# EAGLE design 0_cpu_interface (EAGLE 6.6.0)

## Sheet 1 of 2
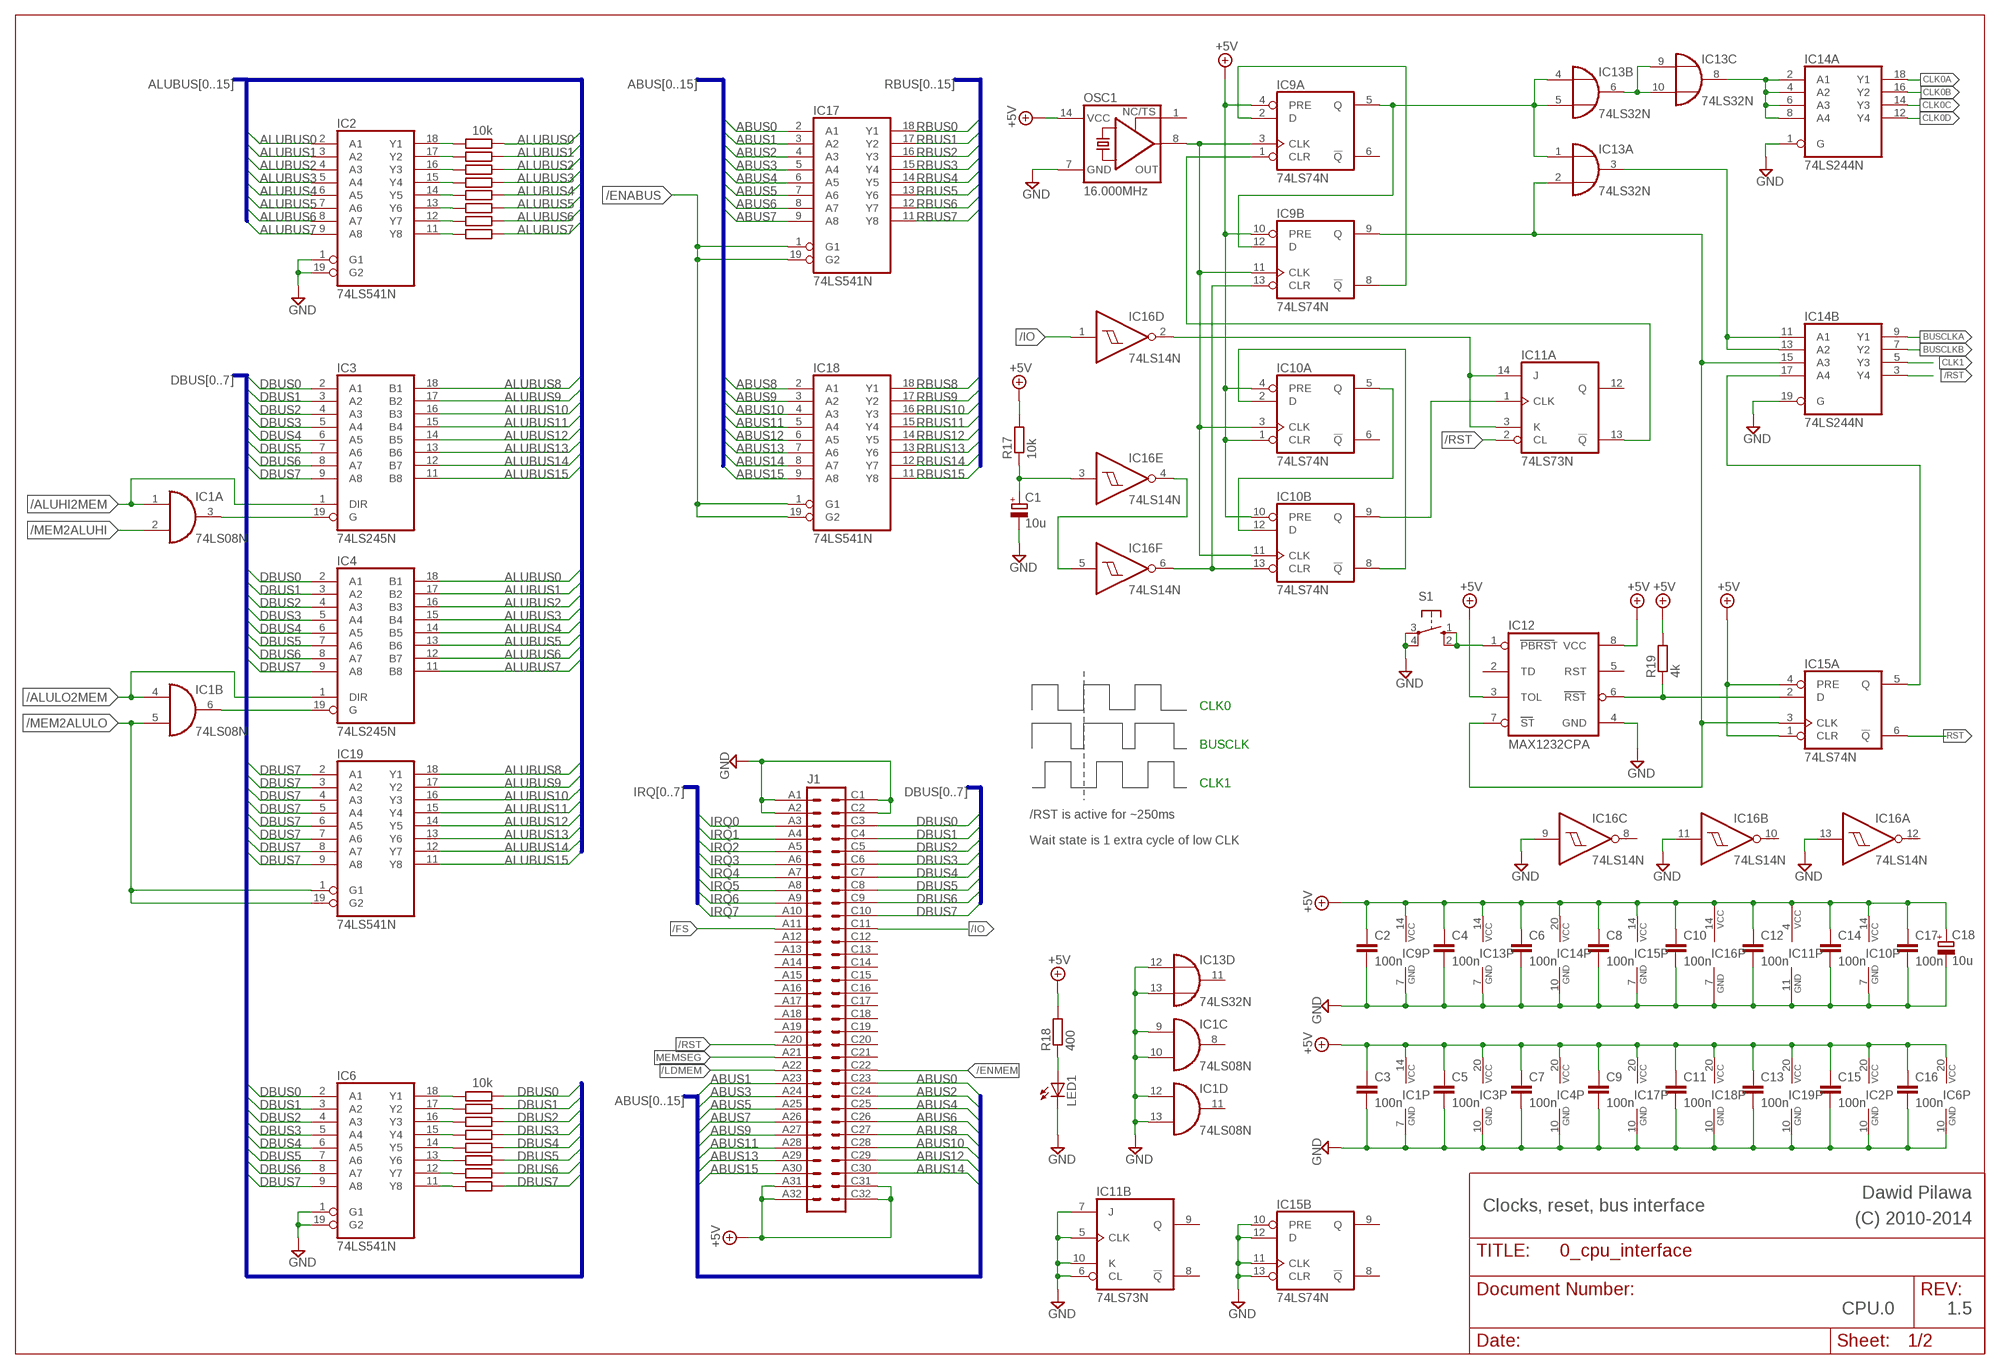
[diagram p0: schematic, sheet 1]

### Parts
C1  10u  CPOL-EUE2.5-5  [E2,5-5]
C2  100n  C-EU050-024X044  [C050-024X044]
C3  100n  C-EU050-024X044  [C050-024X044]
C4  100n  C-EU050-024X044  [C050-024X044]
C5  100n  C-EU050-024X044  [C050-024X044]
C6  100n  C-EU050-024X044  [C050-024X044]
C7  100n  C-EU050-024X044  [C050-024X044]
C8  100n  C-EU050-024X044  [C050-024X044]
C9  100n  C-EU050-024X044  [C050-024X044]
C10  100n  C-EU050-024X044  [C050-024X044]
C11  100n  C-EU050-024X044  [C050-024X044]
C12  100n  C-EU050-024X044  [C050-024X044]
C13  100n  C-EU050-024X044  [C050-024X044]
C14  100n  C-EU050-024X044  [C050-024X044]
C15  100n  C-EU050-024X044  [C050-024X044]
C16  100n  C-EU050-024X044  [C050-024X044]
C17  100n  C-EU050-024X044  [C050-024X044]
C18  10u  CPOL-EUE2.5-6  [E2,5-6]
IC1  74LS08N  [DIL14]
IC2  74LS541N  [DIL20]
IC3  74LS245N  [DIL20]
IC4  74LS245N  [DIL20]
IC6  74LS541N  [DIL20]
IC9  74LS74N  [DIL14]
IC10  74LS74N  [DIL14]
IC11  74LS73N  [DIL14]
IC12  MAX1232CPA  [DIL08]
IC13  74LS32N  [DIL14]
IC14  74LS244N  [DIL20]
IC15  74LS74N  [DIL14]
IC16  74LS14N  [DIL14]
IC17  74LS541N  [DIL20]
IC18  74LS541N  [DIL20]
IC19  74LS541N  [DIL20]
J1  VG64B  [VG64B]
LED1  LED5MM  [LED5MM]
OSC1  16.000MHz  XO-14  [DIL14S]
R1  10k  R-EU_0204/7  [0204/7]
R2  R-EU_0204/7  [0204/7]
R3  R-EU_0204/7  [0204/7]
R4  R-EU_0204/7  [0204/7]
R5  R-EU_0204/7  [0204/7]
R6  R-EU_0204/7  [0204/7]
R7  R-EU_0204/7  [0204/7]
R8  R-EU_0204/7  [0204/7]
R9  10k  R-EU_0204/7  [0204/7]
R10  R-EU_0204/7  [0204/7]
R11  R-EU_0204/7  [0204/7]
R12  R-EU_0204/7  [0204/7]
R13  R-EU_0204/7  [0204/7]
R14  R-EU_0204/7  [0204/7]
R15  R-EU_0204/7  [0204/7]
R16  R-EU_0204/7  [0204/7]
R17  10k  R-EU_0204/7  [0204/7]
R18  400  R-EU_0204/7  [0204/7]
R19  4k  R-EU_0204/7  [0204/7]
S1  10-XX  [B3F-10XX]

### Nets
+5V: C2.1 C3.1 C4.1 C5.1 C6.1 C7.1 C8.1 C9.1 C10.1 C11.1 C12.1 C13.1 C14.1 C15.1 C16.1 C17.1 C18.+ IC1.14(P:VCC) IC2.20(VCC) IC3.20(VCC) IC4.20(VCC) IC6.20(VCC) IC9.4(A:PRE) IC9.10(B:PRE) IC9.14(P:VCC) IC10.1(A:CLR) IC10.4(A:PRE) IC10.10(B:PRE) IC10.14(P:VCC) IC11.4(P:VCC) IC12.3(TOL) IC12.8(VCC) IC13.14(P:VCC) IC14.20(P:VCC) IC15.1(A:CLR) IC15.4(A:PRE) IC15.14(P:VCC) IC16.14(P:VCC) IC17.20(VCC) IC18.20(VCC) IC19.20(VCC) J1.A31 J1.A32 J1.C31 J1.C32 OSC1.14(VCC) R17.2 R18.2 R19.2 ; also sheet 2
/ALUHI2MEM: IC1.1(A:I0) IC3.1(DIR) ; also sheet 2
/ALULO2MEM: IC1.4(B:I0) IC4.1(DIR) ; also sheet 2
/ENABUS: IC17.1(G1) IC17.19(G2) IC18.1(G1) IC18.19(G2) ; also sheet 2
/ENMEM: J1.C22 ; also sheet 2
/FS: J1.A11 ; also sheet 2
/IO: IC16.1(D:I) J1.C11
/LDMEM: J1.A22 ; also sheet 2
/MEM2ALUHI: IC1.2(A:I1) ; also sheet 2
/MEM2ALULO: IC1.5(B:I1) IC19.1(G1) IC19.19(G2) ; also sheet 2
/RST: IC11.2(A:CL) IC14.3(B:Y4) J1.A20 ; also sheet 2
ABUS0: IC17.2(A1) J1.C23 ; also sheet 2
ABUS1: IC17.3(A2) J1.A23 ; also sheet 2
ABUS2: IC17.4(A3) J1.C24 ; also sheet 2
ABUS3: IC17.5(A4) J1.A24 ; also sheet 2
ABUS4: IC17.6(A5) J1.C25 ; also sheet 2
ABUS5: IC17.7(A6) J1.A25 ; also sheet 2
ABUS6: IC17.8(A7) J1.C26 ; also sheet 2
ABUS7: IC17.9(A8) J1.A26 ; also sheet 2
ABUS8: IC18.2(A1) J1.C27 ; also sheet 2
ABUS9: IC18.3(A2) J1.A27 ; also sheet 2
ABUS10: IC18.4(A3) J1.C28 ; also sheet 2
ABUS11: IC18.5(A4) J1.A28 ; also sheet 2
ABUS12: IC18.6(A5) J1.C29 ; also sheet 2
ABUS13: IC18.7(A6) J1.A29 ; also sheet 2
ABUS14: IC18.8(A7) J1.C30 ; also sheet 2
ABUS15: IC18.9(A8) J1.A30 ; also sheet 2
ALUBUS0: IC2.2(A1) IC4.18(B1) R1.2 ; also sheet 2
ALUBUS1: IC2.3(A2) IC4.17(B2) R2.2 ; also sheet 2
ALUBUS2: IC2.4(A3) IC4.16(B3) R3.2 ; also sheet 2
ALUBUS3: IC2.5(A4) IC4.15(B4) R4.2 ; also sheet 2
ALUBUS4: IC2.6(A5) IC4.14(B5) R5.2 ; also sheet 2
ALUBUS5: IC2.7(A6) IC4.13(B6) R6.2 ; also sheet 2
ALUBUS6: IC2.8(A7) IC4.12(B7) R7.2 ; also sheet 2
ALUBUS7: IC2.9(A8) IC4.11(B8) R8.2 ; also sheet 2
ALUBUS8: IC3.18(B1) IC19.18(Y1) ; also sheet 2
ALUBUS9: IC3.17(B2) IC19.17(Y2) ; also sheet 2
ALUBUS10: IC3.16(B3) IC19.16(Y3) ; also sheet 2
ALUBUS11: IC3.15(B4) IC19.15(Y4) ; also sheet 2
ALUBUS12: IC3.14(B5) IC19.14(Y5) ; also sheet 2
ALUBUS13: IC3.13(B6) IC19.13(Y6) ; also sheet 2
ALUBUS14: IC3.12(B7) IC19.12(Y7) ; also sheet 2
ALUBUS15: IC3.11(B8) IC19.11(Y8) ; also sheet 2
BUSCLK: IC13.3(A:O) IC14.11(B:A1) IC14.13(B:A2)
BUSCLKA: IC14.9(B:Y1) ; also sheet 2
BUSCLKB: IC14.7(B:Y2) ; also sheet 2
CLK0: IC9.5(A:Q) IC9.12(B:D) IC13.1(A:I0) IC13.4(B:I0) IC13.5(B:I1)
CLK0A: IC14.18(A:Y1) ; also sheet 2
CLK0B: IC14.16(A:Y2) ; also sheet 2
CLK0C: IC14.14(A:Y3) ; also sheet 2
CLK0D: IC14.12(A:Y4) ; also sheet 2
CLK1: IC14.5(B:Y3) ; also sheet 2
DBUS0: IC3.2(A1) IC4.2(A1) IC6.2(A1) J1.C3 R9.2 ; also sheet 2
DBUS1: IC3.3(A2) IC4.3(A2) IC6.3(A2) J1.C4 R10.2 ; also sheet 2
DBUS2: IC3.4(A3) IC4.4(A3) IC6.4(A3) J1.C5 R11.2 ; also sheet 2
DBUS3: IC3.5(A4) IC4.5(A4) IC6.5(A4) J1.C6 R12.2 ; also sheet 2
DBUS4: IC3.6(A5) IC4.6(A5) IC6.6(A5) J1.C7 R13.2 ; also sheet 2
DBUS5: IC3.7(A6) IC4.7(A6) IC6.7(A6) J1.C8 R14.2 ; also sheet 2
DBUS6: IC3.8(A7) IC4.8(A7) IC6.8(A7) J1.C9 R15.2 ; also sheet 2
DBUS7: IC3.9(A8) IC4.9(A8) IC6.9(A8) IC19.2(A1) IC19.3(A2) IC19.4(A3) IC19.5(A4) IC19.6(A5) IC19.7(A6) IC19.8(A7) IC19.9(A8) J1.C10 R16.2 ; also sheet 2
GND: C1.- C2.2 C3.2 C4.2 C5.2 C6.2 C7.2 C8.2 C9.2 C10.2 C11.2 C12.2 C13.2 C14.2 C15.2 C16.2 C17.2 C18.- IC1.7(P:GND) IC1.9(C:I0) IC1.10(C:I1) IC1.12(D:I0) IC1.13(D:I1) IC2.1(G1) IC2.10(GND) IC2.19(G2) IC3.10(GND) IC4.10(GND) IC6.1(G1) IC6.10(GND) IC6.19(G2) IC9.7(P:GND) IC10.7(P:GND) IC11.5(B:CLK) IC11.6(B:CL) IC11.7(B:J) IC11.10(B:K) IC11.11(P:GND) IC12.4(GND) IC13.7(P:GND) IC13.12(D:I0) IC13.13(D:I1) IC14.1(A:G) IC14.10(P:GND) IC14.19(B:G) IC15.7(P:GND) IC15.10(B:PRE) IC15.11(B:CLK) IC15.12(B:D) IC15.13(B:CLR) IC16.7(P:GND) IC16.9(C:I) IC16.11(B:I) IC16.13(A:I) IC17.10(GND) IC18.10(GND) IC19.10(GND) J1.A1 J1.A2 J1.C1 J1.C2 LED1.K(C) OSC1.7(GND) S1.3(P) S1.4(P1) ; also sheet 2
IRQ0: J1.A3 ; also sheet 2
IRQ1: J1.A4 ; also sheet 2
IRQ2: J1.A5 ; also sheet 2
IRQ3: J1.A6 ; also sheet 2
IRQ4: J1.A7 ; also sheet 2
IRQ5: J1.A8 ; also sheet 2
IRQ6: J1.A9 ; also sheet 2
IRQ7: J1.A10 ; also sheet 2
MEMSEG: J1.A21 ; also sheet 2
N$1: IC1.3(A:O) IC3.19(G)
N$2: IC1.6(B:O) IC4.19(G)
N$3: IC2.18(Y1) R1.1
N$4: IC2.17(Y2) R2.1
N$5: IC2.16(Y3) R3.1
N$6: IC2.15(Y4) R4.1
N$7: IC2.14(Y5) R5.1
N$8: IC2.13(Y6) R6.1
N$9: IC2.12(Y7) R7.1
N$10: IC2.11(Y8) R8.1
N$11: IC6.18(Y1) R9.1
N$12: IC6.17(Y2) R10.1
N$13: IC6.16(Y3) R11.1
N$14: IC6.15(Y4) R12.1
N$15: IC6.14(Y5) R13.1
N$16: IC6.12(Y7) R15.1
N$17: IC6.11(Y8) R16.1
N$18: IC6.13(Y6) R14.1
N$19: IC12.1(PBRST) S1.1(S) S1.2(S1)
N$20: IC9.3(A:CLK) IC9.11(B:CLK) IC10.3(A:CLK) IC10.11(B:CLK) OSC1.8(OUT)
N$21: LED1.A R18.1
N$22: IC9.2(A:D) IC9.8(B:!Q)
N$23: IC14.17(B:A4) IC15.5(A:Q)
N$24: IC12.6(RST) IC15.2(A:D) R19.1
N$25: IC10.2(A:D) IC10.8(B:!Q)
N$26: IC13.8(C:O) IC14.2(A:A1) IC14.4(A:A2) IC14.6(A:A3) IC14.8(A:A4)
N$27: IC9.1(A:CLR) IC11.13(A:!Q)
N$28: C1.+ IC16.3(E:I) R17.1
N$29: IC13.6(B:O) IC13.9(C:I0) IC13.10(C:I1)
N$30: IC9.9(B:Q) IC12.7(ST) IC13.2(A:I1) IC14.15(B:A3) IC15.3(A:CLK)
N$31: IC10.5(A:Q) IC10.12(B:D)
N$32: IC10.9(B:Q) IC11.1(A:CLK)
N$33: IC11.3(A:K) IC11.14(A:J) IC16.2(D:O)
N$34: IC16.4(E:O) IC16.5(F:I)
N$35: IC9.13(B:CLR) IC10.13(B:CLR) IC16.6(F:O)
RBUS0: IC17.18(Y1) ; also sheet 2
RBUS1: IC17.17(Y2) ; also sheet 2
RBUS2: IC17.16(Y3) ; also sheet 2
RBUS3: IC17.15(Y4) ; also sheet 2
RBUS4: IC17.14(Y5) ; also sheet 2
RBUS5: IC17.13(Y6) ; also sheet 2
RBUS6: IC17.12(Y7) ; also sheet 2
RBUS7: IC17.11(Y8) ; also sheet 2
RBUS8: IC18.18(Y1) ; also sheet 2
RBUS9: IC18.17(Y2) ; also sheet 2
RBUS10: IC18.16(Y3) ; also sheet 2
RBUS11: IC18.15(Y4) ; also sheet 2
RBUS12: IC18.14(Y5) ; also sheet 2
RBUS13: IC18.13(Y6) ; also sheet 2
RBUS14: IC18.12(Y7) ; also sheet 2
RBUS15: IC18.11(Y8) ; also sheet 2
RST: IC15.6(A:!Q) ; also sheet 2
Unconnected: IC1.8(C:O) IC1.11(D:O) IC9.6(A:!Q) IC10.6(A:!Q) IC11.8(B:!Q) IC11.9(B:Q) IC11.12(A:Q) IC12.2(TD) IC12.5(RST) IC13.11(D:O) IC15.8(B:!Q) IC15.9(B:Q) IC16.8(C:O) IC16.10(B:O) IC16.12(A:O) J1.A12 J1.A13 J1.A14 J1.A15 J1.A16 J1.A17 J1.A18 J1.A19 J1.C12 J1.C13 J1.C14 J1.C15 J1.C16 J1.C17 J1.C18 J1.C19 J1.C20 J1.C21 OSC1.1(TS)

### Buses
DBUS[0..7]
ALUBUS[0..15]
RBUS[0..15]
IRQ[0..7]
ABUS[0..15]

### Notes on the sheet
- CLK0
- BUSCLK
- CLK1
- /RST is active for ~250ms
- Wait state is 1 extra cycle of low CLK
- Dawid Pilawa
- Clocks, reset, bus interface | (C) 2010-2014
- CPU.0 | 1.5

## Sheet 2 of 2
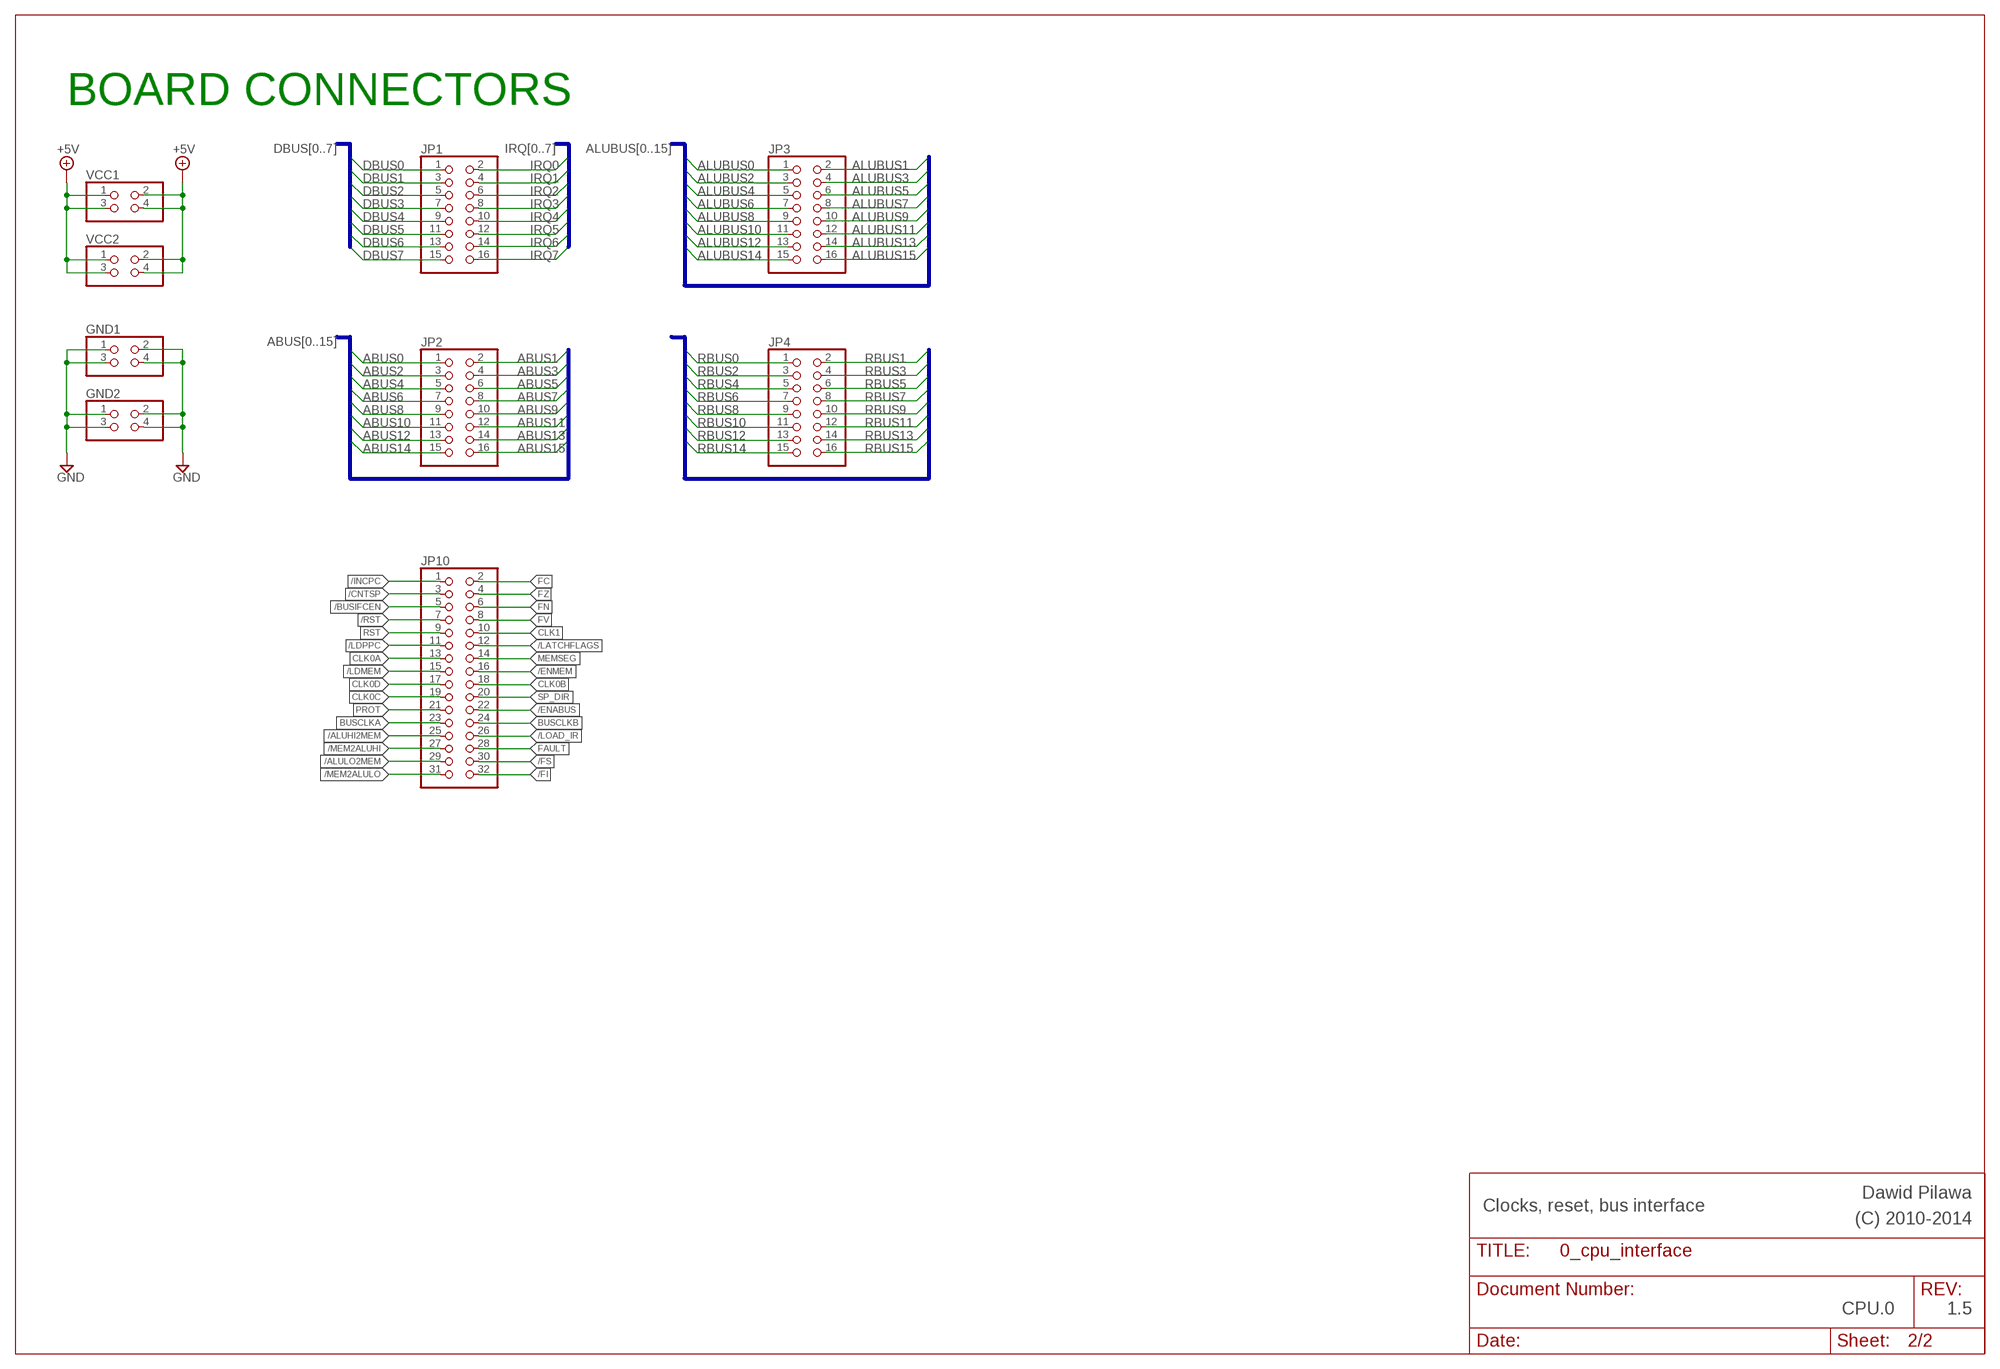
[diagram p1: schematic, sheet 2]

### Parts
GND1  PINHD-2X2  [2X02]
GND2  PINHD-2X2  [2X02]
JP1  PINHD-2X8  [2X08]
JP2  PINHD-2X8  [2X08]
JP3  PINHD-2X8  [2X08]
JP4  PINHD-2X8  [2X08]
JP10  PINHD-2X16  [2X16]
VCC1  PINHD-2X2  [2X02]
VCC2  PINHD-2X2  [2X02]

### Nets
+5V: VCC1.1 VCC1.2 VCC1.3 VCC1.4 VCC2.1 VCC2.2 VCC2.3 VCC2.4 ; also sheet 1
/ALUHI2MEM: JP10.25 ; also sheet 1
/ALULO2MEM: JP10.29 ; also sheet 1
/BUSIFCEN: JP10.5
/CNTSP: JP10.3
/ENABUS: JP10.22 ; also sheet 1
/ENMEM: JP10.16 ; also sheet 1
/FI: JP10.32
/FS: JP10.30 ; also sheet 1
/INCPC: JP10.1
/LATCHFLAGS: JP10.12
/LDMEM: JP10.15 ; also sheet 1
/LDPPC: JP10.11
/LOAD_IR: JP10.26
/MEM2ALUHI: JP10.27 ; also sheet 1
/MEM2ALULO: JP10.31 ; also sheet 1
/RST: JP10.7 ; also sheet 1
ABUS0: JP2.1 ; also sheet 1
ABUS1: JP2.2 ; also sheet 1
ABUS2: JP2.3 ; also sheet 1
ABUS3: JP2.4 ; also sheet 1
ABUS4: JP2.5 ; also sheet 1
ABUS5: JP2.6 ; also sheet 1
ABUS6: JP2.7 ; also sheet 1
ABUS7: JP2.8 ; also sheet 1
ABUS8: JP2.9 ; also sheet 1
ABUS9: JP2.10 ; also sheet 1
ABUS10: JP2.11 ; also sheet 1
ABUS11: JP2.12 ; also sheet 1
ABUS12: JP2.13 ; also sheet 1
ABUS13: JP2.14 ; also sheet 1
ABUS14: JP2.15 ; also sheet 1
ABUS15: JP2.16 ; also sheet 1
ALUBUS0: JP3.1 ; also sheet 1
ALUBUS1: JP3.2 ; also sheet 1
ALUBUS2: JP3.3 ; also sheet 1
ALUBUS3: JP3.4 ; also sheet 1
ALUBUS4: JP3.5 ; also sheet 1
ALUBUS5: JP3.6 ; also sheet 1
ALUBUS6: JP3.7 ; also sheet 1
ALUBUS7: JP3.8 ; also sheet 1
ALUBUS8: JP3.9 ; also sheet 1
ALUBUS9: JP3.10 ; also sheet 1
ALUBUS10: JP3.11 ; also sheet 1
ALUBUS11: JP3.12 ; also sheet 1
ALUBUS12: JP3.13 ; also sheet 1
ALUBUS13: JP3.14 ; also sheet 1
ALUBUS14: JP3.15 ; also sheet 1
ALUBUS15: JP3.16 ; also sheet 1
BUSCLKA: JP10.23 ; also sheet 1
BUSCLKB: JP10.24 ; also sheet 1
CLK0A: JP10.13 ; also sheet 1
CLK0B: JP10.18 ; also sheet 1
CLK0C: JP10.19 ; also sheet 1
CLK0D: JP10.17 ; also sheet 1
CLK1: JP10.10 ; also sheet 1
DBUS0: JP1.1 ; also sheet 1
DBUS1: JP1.3 ; also sheet 1
DBUS2: JP1.5 ; also sheet 1
DBUS3: JP1.7 ; also sheet 1
DBUS4: JP1.9 ; also sheet 1
DBUS5: JP1.11 ; also sheet 1
DBUS6: JP1.13 ; also sheet 1
DBUS7: JP1.15 ; also sheet 1
FAULT: JP10.28
FC: JP10.2
FN: JP10.6
FV: JP10.8
FZ: JP10.4
GND: GND1.1 GND1.2 GND1.3 GND1.4 GND2.1 GND2.2 GND2.3 GND2.4 ; also sheet 1
IRQ0: JP1.2 ; also sheet 1
IRQ1: JP1.4 ; also sheet 1
IRQ2: JP1.6 ; also sheet 1
IRQ3: JP1.8 ; also sheet 1
IRQ4: JP1.10 ; also sheet 1
IRQ5: JP1.12 ; also sheet 1
IRQ6: JP1.14 ; also sheet 1
IRQ7: JP1.16 ; also sheet 1
MEMSEG: JP10.14 ; also sheet 1
PROT: JP10.21
RBUS0: JP4.1 ; also sheet 1
RBUS1: JP4.2 ; also sheet 1
RBUS2: JP4.3 ; also sheet 1
RBUS3: JP4.4 ; also sheet 1
RBUS4: JP4.5 ; also sheet 1
RBUS5: JP4.6 ; also sheet 1
RBUS6: JP4.7 ; also sheet 1
RBUS7: JP4.8 ; also sheet 1
RBUS8: JP4.9 ; also sheet 1
RBUS9: JP4.10 ; also sheet 1
RBUS10: JP4.11 ; also sheet 1
RBUS11: JP4.12 ; also sheet 1
RBUS12: JP4.13 ; also sheet 1
RBUS13: JP4.14 ; also sheet 1
RBUS14: JP4.15 ; also sheet 1
RBUS15: JP4.16 ; also sheet 1
RST: JP10.9 ; also sheet 1
SP_DIR: JP10.20

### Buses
DBUS[0..7]
ALUBUS[0..15]
RBUS[0..15]
IRQ[0..7]
ABUS[0..15]

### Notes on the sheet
- BOARD CONNECTORS
- Dawid Pilawa
- Clocks, reset, bus interface | (C) 2010-2014
- CPU.0 | 1.5

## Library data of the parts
C1 C18 = rcl:CPOL-EU: POLARIZED CAPACITOR, European symbol
C2-C17 = rcl:C-EU: CAPACITOR, European symbol
GND1 GND2 VCC1 VCC2 = pinhead:PINHD-2X2: PIN HEADER
IC1 = 74xx-eu:74*08: Quad 2-input AND gate
IC2 IC6 IC17-IC19 = 74xx-eu:74*541: Octal BUFFER and LINE DRIVER, 3-state
IC3 IC4 = 74xx-eu:74*245: Octal BUS TRANSCEIVER, 3-state
IC9 IC10 IC15 = 74xx-eu:74*74: Dual D type positive edge triggered FLIP FLOP, preset and clear
IC11 = 74xx-us:74*73: Dual J-K FLIP FLOP, clear
IC12 = maxim:MAX1232CPA: MONITOR DEVICE
IC13 = 74xx-eu:74*32: Quad 2-input OR gate
IC14 = 74xx-eu:74*244: Octal BUFFER and LINE DRIVER, 3-state
IC16 = 74xx-us:74*14: Hex schmitt trigger INVERTER
J1 = 19inch:VG64: PCB EUROCARD, 64-pin type C/AC, 2.54 mm
JP1-JP4 = pinhead:PINHD-2X8: PIN HEADER
JP10 = pinhead:PINHD-2X16: PIN HEADER
LED1 = led:LED: LED
OSC1 = crystal:XO-: CRYSTAL
R1-R19 = rcl:R-EU_: RESISTOR, European symbol
S1 = switch-omron:10-XX: OMRON SWITCH

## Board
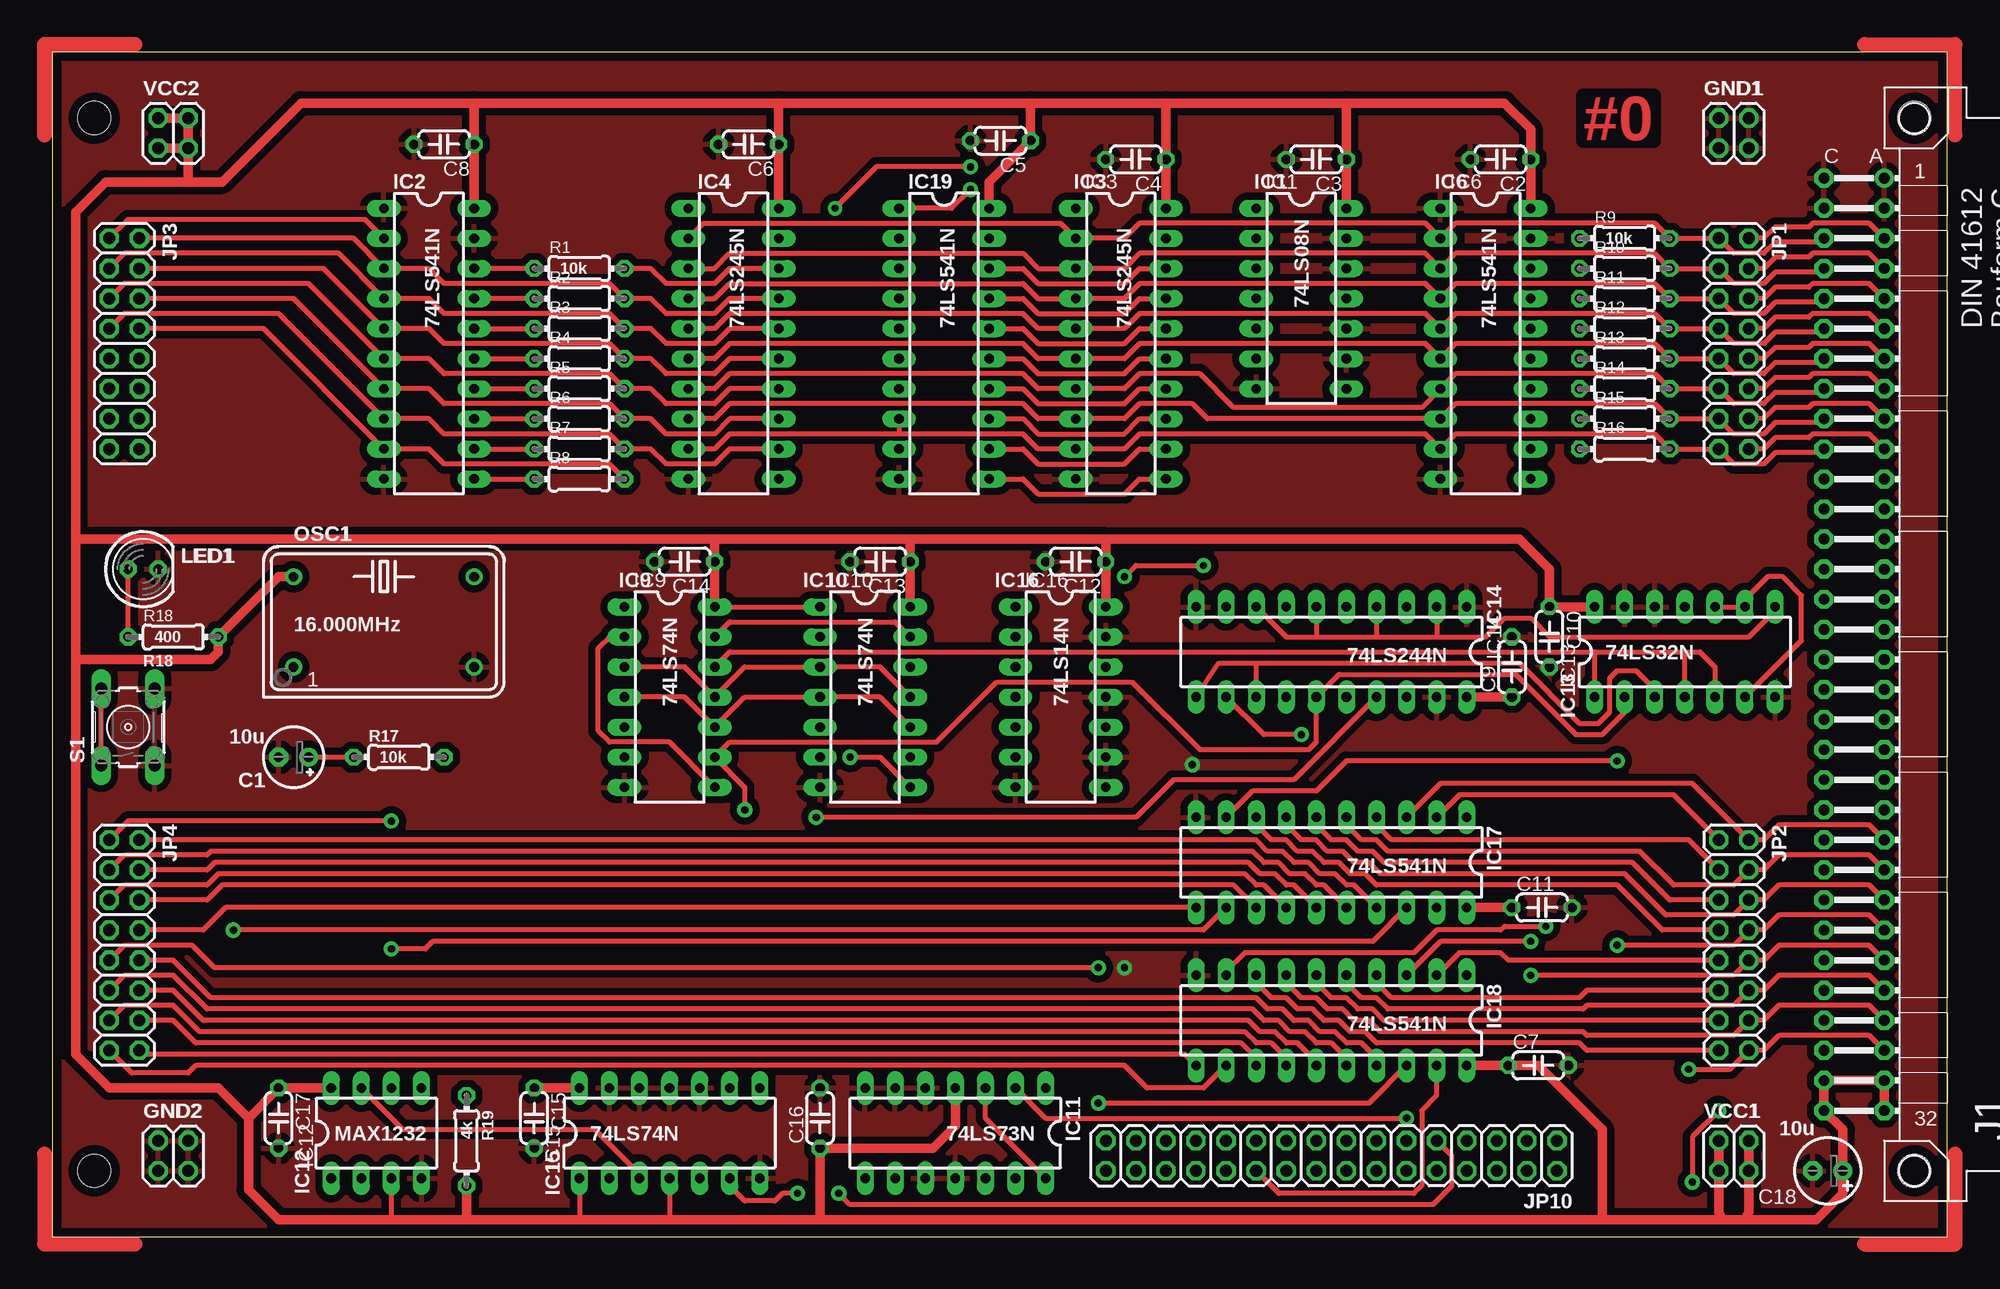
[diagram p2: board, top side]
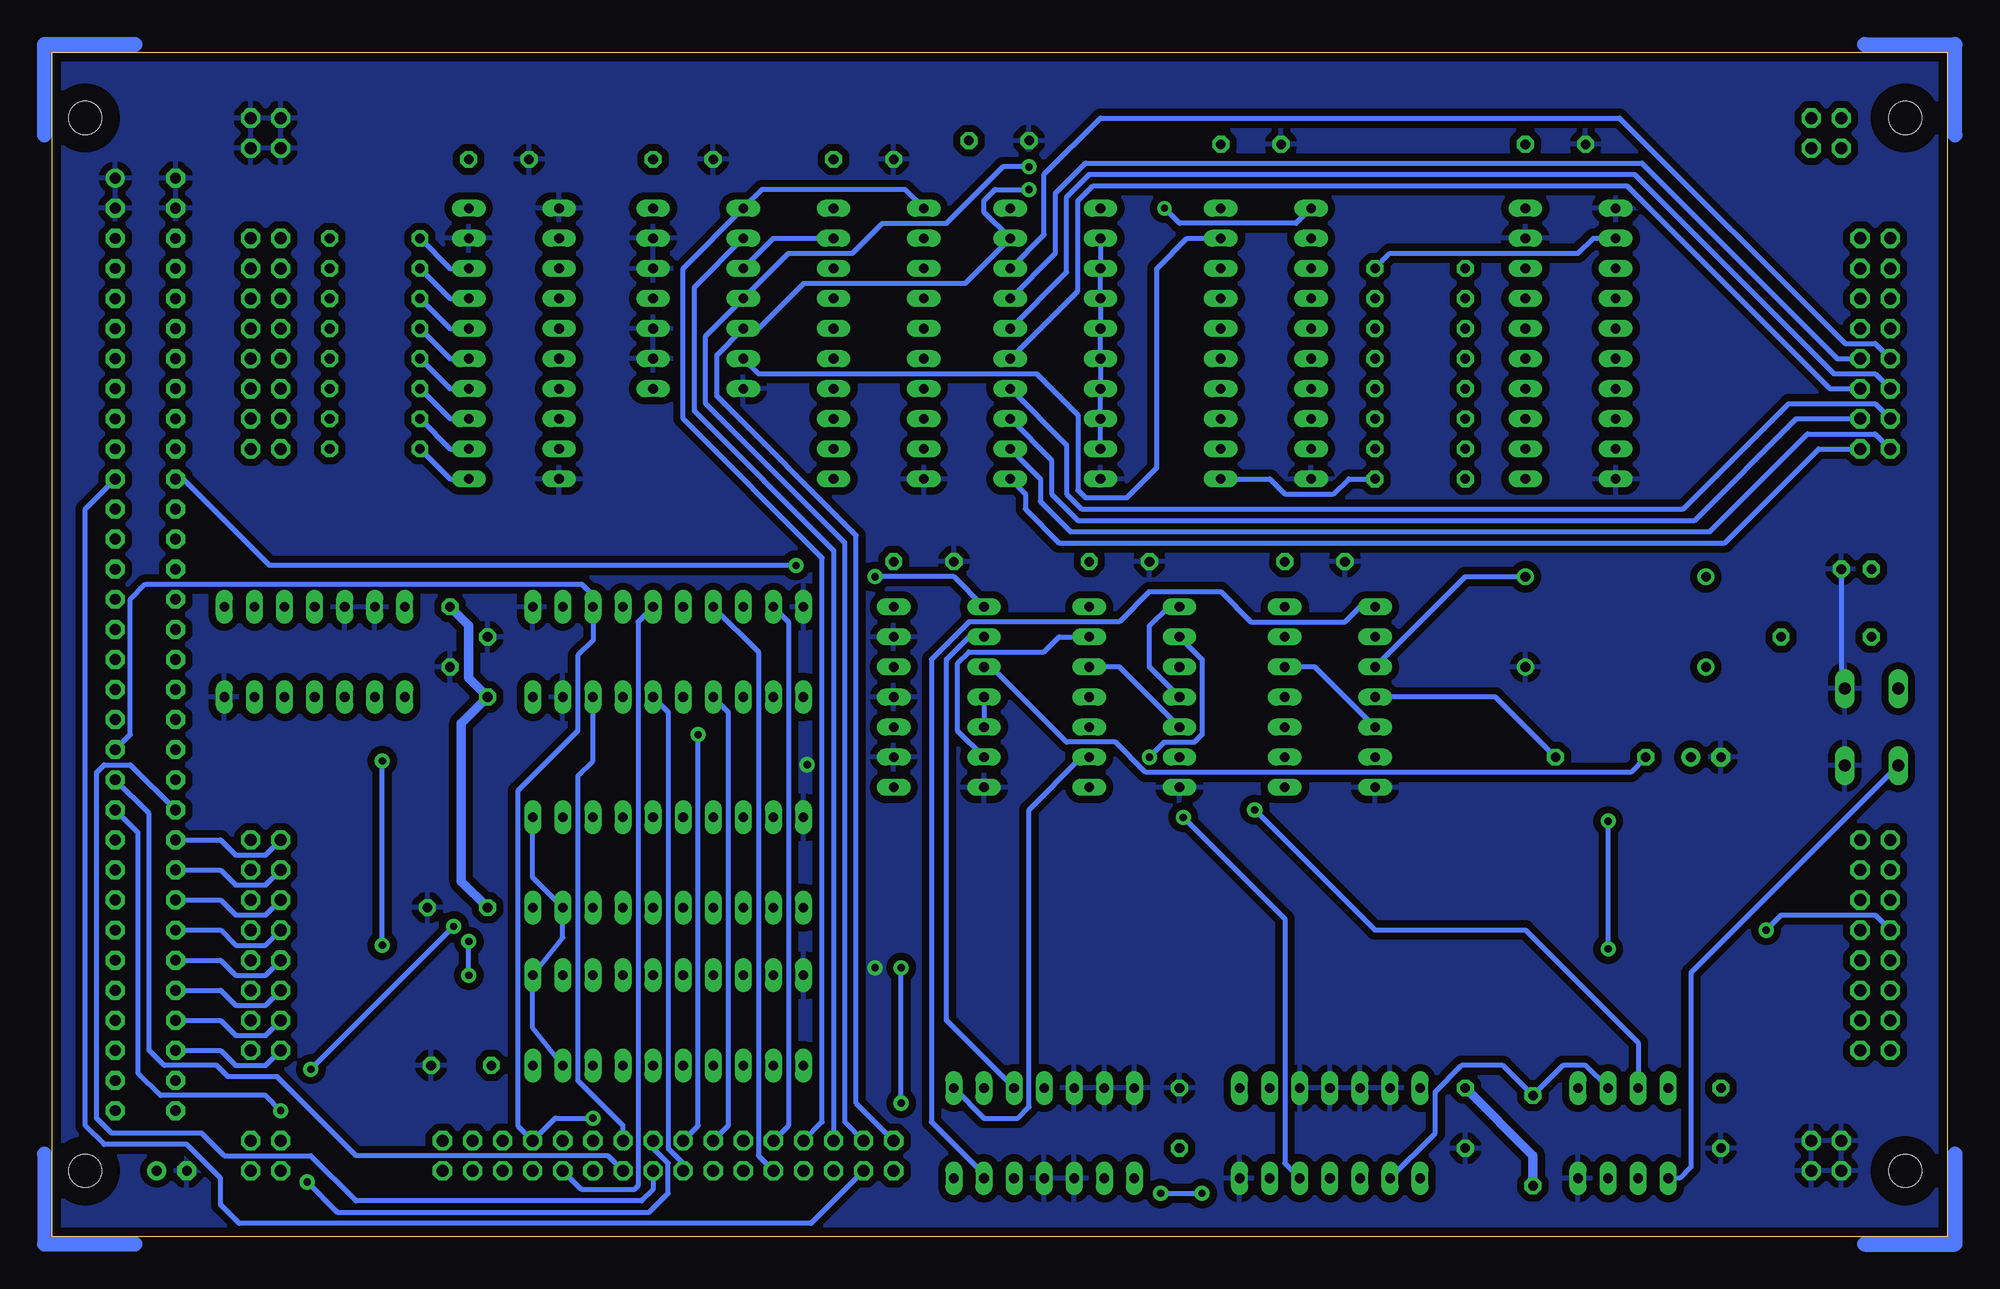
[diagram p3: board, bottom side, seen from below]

Size 160.02 x 100.03 mm. Coordinates in mm from the lower left corner, seen from the top.
Copper layers (1*16): Top 0.035mm / dielectric 1.5mm / Bottom 0.035mm
Design rules "homebrew_pcb": minimum track width 16mil, minimum drill 24mil, track to track 16mil, track to pad 10mil, pad to pad 10mil, via to via 10mil, smd to smd 8mil, copper to edge 30mil, drill to drill 10mil, minimum pad ring 12mil, minimum via ring 12mil, stop-mask expansion 4mil, vias tented up to drill 0mil, thermal gap 24mil

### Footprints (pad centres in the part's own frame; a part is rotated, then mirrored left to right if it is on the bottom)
E2,5-5 = drill 0.813 pad 1.6: + -1.27,0 | drill 0.813 pad 1.6 octagon: - 1.27,0
C050-024X044 = drill 0.813 octagon: 1 -2.54,0; 2 2.54,0
E2,5-6 = drill 0.813 pad 1.6: + -1.27,0 | drill 0.813 pad 1.6 octagon: - 1.27,0
2X02 = drill 1.016 octagon: 1 -1.27,-1.27; 2 -1.27,1.27; 3 1.27,-1.27; 4 1.27,1.27
DIL14 = drill 0.813 long: 1 -7.62,-3.81; 2 -5.08,-3.81; 3 -2.54,-3.81; 4 0,-3.81; 5 2.54,-3.81; 6 5.08,-3.81; 7 7.62,-3.81; 8 7.62,3.81; 9 5.08,3.81; 10 2.54,3.81; 11 0,3.81; 12 -2.54,3.81; 13 -5.08,3.81; 14 -7.62,3.81
DIL20 = drill 0.813 long: 1 -11.43,-3.81; 2 -8.89,-3.81; 3 -6.35,-3.81; 4 -3.81,-3.81; 5 -1.27,-3.81; 6 1.27,-3.81; 7 3.81,-3.81; 8 6.35,-3.81; 9 8.89,-3.81; 10 11.43,-3.81; 11 11.43,3.81; 12 8.89,3.81; 13 6.35,3.81; 14 3.81,3.81; 15 1.27,3.81; 16 -1.27,3.81; 17 -3.81,3.81; 18 -6.35,3.81; 19 -8.89,3.81; 20 -11.43,3.81
DIL08 = drill 0.813 long: 1 -3.81,-3.81; 2 -1.27,-3.81; 3 1.27,-3.81; 4 3.81,-3.81; 5 3.81,3.81; 6 1.27,3.81; 7 -1.27,3.81; 8 -3.81,3.81
VG64B = drill 0.914 pad 1.6: A1 154.94,39.37 | drill 0.914 pad 1.6 octagon: A2 154.94,36.83; A3 154.94,34.29; A4 154.94,31.75; A5 154.94,29.21; A6 154.94,26.67; A7 154.94,24.13; A8 154.94,21.59; A9 154.94,19.05; A10 154.94,16.51; A11 154.94,13.97; A12 154.94,11.43; A13 154.94,8.89; A14 154.94,6.35; A15 154.94,3.81; A16 154.94,1.27; A17 154.94,-1.27; A18 154.94,-3.81; A19 154.94,-6.35; A20 154.94,-8.89; A21 154.94,-11.43; A22 154.94,-13.97; A23 154.94,-16.51; A24 154.94,-19.05; A25 154.94,-21.59; A26 154.94,-24.13; A27 154.94,-26.67; A28 154.94,-29.21; A29 154.94,-31.75; A30 154.94,-34.29; A31 154.94,-36.83; A32 154.94,-39.37; C1 149.86,39.37; C2 149.86,36.83; C3 149.86,34.29; C4 149.86,31.75; C5 149.86,29.21; C6 149.86,26.67; C7 149.86,24.13; C8 149.86,21.59; C9 149.86,19.05; C10 149.86,16.51; C11 149.86,13.97; C12 149.86,11.43; C13 149.86,8.89; C14 149.86,6.35; C15 149.86,3.81; C16 149.86,1.27; C17 149.86,-1.27; C18 149.86,-3.81; C19 149.86,-6.35; C20 149.86,-8.89; C21 149.86,-11.43; C22 149.86,-13.97; C23 149.86,-16.51; C24 149.86,-19.05; C25 149.86,-21.59; C26 149.86,-24.13; C27 149.86,-26.67; C28 149.86,-29.21; C29 149.86,-31.75; C30 149.86,-34.29; C31 149.86,-36.83; C32 149.86,-39.37 | hole 2.794: 157.48,44.45; 157.48,-44.45; 3.81,-44.45; 3.81,44.45
2X08 = drill 1.016 octagon: 1 -8.89,-1.27; 2 -8.89,1.27; 3 -6.35,-1.27; 4 -6.35,1.27; 5 -3.81,-1.27; 6 -3.81,1.27; 7 -1.27,-1.27; 8 -1.27,1.27; 9 1.27,-1.27; 10 1.27,1.27; 11 3.81,-1.27; 12 3.81,1.27; 13 6.35,-1.27; 14 6.35,1.27; 15 8.89,-1.27; 16 8.89,1.27
2X16 = drill 1.016 octagon: 1 -19.05,-1.27; 2 -19.05,1.27; 3 -16.51,-1.27; 4 -16.51,1.27; 5 -13.97,-1.27; 6 -13.97,1.27; 7 -11.43,-1.27; 8 -11.43,1.27; 9 -8.89,-1.27; 10 -8.89,1.27; 11 -6.35,-1.27; 12 -6.35,1.27; 13 -3.81,-1.27; 14 -3.81,1.27; 15 -1.27,-1.27; 16 -1.27,1.27; 17 1.27,-1.27; 18 1.27,1.27; 19 3.81,-1.27; 20 3.81,1.27; 21 6.35,-1.27; 22 6.35,1.27; 23 8.89,-1.27; 24 8.89,1.27; 25 11.43,-1.27; 26 11.43,1.27; 27 13.97,-1.27; 28 13.97,1.27; 29 16.51,-1.27; 30 16.51,1.27; 31 19.05,-1.27; 32 19.05,1.27
LED5MM = drill 0.813 octagon: A -1.27,0; K 1.27,0
DIL14S = drill 0.813: 1 -7.62,-3.81; 7 7.62,-3.81; 8 7.62,3.81; 14 -7.62,3.81
0204/7 = drill 0.813 octagon: 1 -3.81,0; 2 3.81,0
B3F-10XX = drill 1.016 long: 1 -3.251,2.261; 2 3.251,2.261; 3 -3.251,-2.261; 4 3.251,-2.261

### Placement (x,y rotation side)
C1  20.38,40.49 180 top
C2  122.3,90.97 180 top
C3  106.74,90.97 180 top
C4  91.5,90.97 180 top
C5  80.07,92.56 180 top
C6  58.8,92.24 180 top
C7  125.48,14.45 0 top
C8  33.08,92.24 180 top
C9  123.25,48.11 90 top
C10  126.43,50.65 270 top
C11  125.79,27.79 0 top
C12  86.42,57 180 top
C13  69.91,57 180 top
C14  53.4,57 180 top
C15  40.7,10.01 270 top
C16  64.83,10.01 90 top
C17  19.11,10.01 270 top
C18  149.92,5.56 180 top
GND1  141.99,93.19 0 top
GND2  10.22,6.83 0 top
IC1  105.47,79.22 270 top
IC2  31.81,75.41 270 top
IC3  90.23,75.41 270 top
IC4  57.53,75.41 270 top
IC6  121.03,75.41 270 top
IC9  52.13,45.57 270 top
IC10  68.64,45.57 270 top
IC11  76.26,8.74 180 top
IC12  27.37,8.74 0 top
IC13  137.86,49.38 0 top
IC14  108.01,49.38 180 top
IC15  52.13,8.74 0 top
IC16  85.15,45.57 270 top
IC17  108.01,31.6 180 top
IC18  108.01,18.26 180 top
IC19  75.31,75.41 270 top
J1  -0.25,50.01 0 top
JP1  141.99,75.41 270 top
JP2  141.99,24.61 270 top
JP3  6.1,75.41 270 top
JP4  6.1,24.61 270 top
JP10  108.01,6.83 180 top
LED1  7.68,56.36 0 top
OSC1  28,51.92 0 top
R1  44.51,81.76 0 top
R2  44.51,79.22 0 top
R3  44.51,76.68 0 top
R4  44.51,74.14 0 top
R5  44.51,71.6 0 top
R6  44.51,69.06 0 top
R7  44.51,66.52 0 top
R8  44.51,63.98 0 top
R9  132.78,84.3 0 top
R10  132.78,81.76 0 top
R11  132.78,79.22 0 top
R12  132.78,76.68 0 top
R13  132.78,74.14 0 top
R14  132.78,71.6 0 top
R15  132.78,69.06 0 top
R16  132.78,66.52 0 top
R17  29.27,40.49 0 top
R18  10.22,50.65 0 top
R19  34.99,8.1 270 top
S1  6.41,43.03 90 top
VCC1  141.99,6.83 0 top
VCC2  10.22,93.19 0 top

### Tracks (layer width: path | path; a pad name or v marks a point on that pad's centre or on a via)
+5V
  Top 0.406: IC12.3 28.64,1.43 | IC15.1 44.51,1.43 | IC15.4 52.13,1.43 | IC10.10 69.91,45.57 IC10.4 58.48,45.57 IC9.10 53.4,45.57 IC9.4 | IC9.14 IC10.1
  Top 0.813: 130.87,1.43 64.83,1.43 | 64.83,1.43 52.13,1.43 44.51,1.43 34.99,1.43 | 34.99,1.43 28.64,1.43 19.11,1.43 16.57,3.98 16.57,10.01 | 1.97,48.74 1.97,58.9 | 1.97,58.9 1.97,86.52 4.51,89.07 11.49,89.07 | 35.62,95.73 21.02,95.73 14.35,89.07 11.49,89.07 | 35.62,95.73 61.34,95.73 | 61.34,95.73 82.61,95.73 | 82.61,95.73 94.04,95.73 | 94.04,95.73 109.28,95.73 | 109.28,95.73 122.62,95.73 124.84,93.51 C2.1 IC6.20 | 109.28,95.73 C3.1 IC1.14 | 94.04,95.73 C4.1 IC3.20 | 88.96,58.9 72.45,58.9 | 72.45,58.9 55.94,58.9 | 55.94,58.9 1.97,58.9 | 88.96,58.9 C12.1 IC16.14 | 72.45,58.9 C13.1 IC10.14 | 55.94,58.9 C14.1 IC9.14 | OSC1.14 19.11,55.73 R18.2 14.03,49.38 13.4,48.74 1.97,48.74 | IC15.14 C15.1 | IC12.8 C17.1 16.57,10.01 | 64.83,1.43 C16.1 74.36,7.47 76.26,9.37 IC11.4 | 1.97,48.74 1.97,15.4 4.83,12.55 14.03,12.55 16.57,10.01 | 88.96,58.9 123.89,58.9 126.43,56.36 C10.1 IC13.14 | 130.87,1.43 130.87,9.05 125.48,14.45 C7.1 IC18.20 | 130.87,1.43 141.03,1.43 | 141.03,1.43 142.94,1.43 | 142.94,1.43 148.97,1.43 151.19,3.66 C18.+ 151.19,9.05 J1.C32 J1.C31 J1.A31 J1.A32 | 142.94,1.43 143.26,2.07 VCC1.3 VCC1.4 | 141.03,1.43 140.72,2.07 VCC1.1 VCC1.2 | IC14.20 C9.1 | IC4.20 C6.1 61.34,95.73 | IC2.20 C8.1 35.62,95.73 | R19.2 34.99,1.43 | C11.1 IC17.20 | VCC2.3 11.49,89.07 | VCC2.3 VCC2.1 | VCC2.3 VCC2.4 VCC2.2 | IC19.20 79.12,89.07 C5.1 82.61,95.73
  Bottom 0.406: R17.2 38.16,45.57 IC9.4 | IC10.4 67.37,48.11 67.37,51.6 65.79,53.19 IC10.1
  Bottom 0.813: C11.1 125.48,30.01 125.48,43.35 C9.1 124.84,47.15 124.84,51.6 C10.1 | C15.1 34.99,6.83 R19.2
/ALUHI2MEM
  Bottom 0.406: IC3.1 88.01,88.43 100.08,88.43 IC1.1 106.74,81.76 106.74,69.06 95,57.32 95,9.69 JP10.25
/ALULO2MEM  (via drill 0.61 pad 1.02, 0.61 pad 1.27)
  Top 0.406: v77.53,90.33 69.6,90.33 v66.1,86.84
  Bottom 0.406: v77.53,90.33 79.76,90.33 84.52,85.57 89.92,85.57 92.46,83.03 97.85,83.03 IC1.4 104.84,76.05 104.84,70.33 93.09,58.58 93.09,9.69 JP10.29 | IC4.1 54.99,85.57 64.83,85.57 v66.1,86.84
/ENABUS
  Top 0.406: IC18.19 116.9,11.91 115.63,10.64 115.63,4.29 115,3.66 103.57,3.66 JP10.22
  Bottom 0.406: IC18.19 119.44,17.63 IC18.1 116.9,25.25 IC17.19 119.44,30.33 IC17.1
/ENMEM
  Bottom 0.406: J1.C22 153.42,39.85 155.64,39.85 156.27,39.22 156.27,10.01 155,8.74 147.38,8.74 145.48,6.83 138.18,6.83 134.37,3.02 110.24,3.02 109.28,3.98 JP10.16
/FS
  Bottom 0.406: J1.A11 157.23,61.44 157.23,9.37 155.64,7.79 148.65,7.79 145.8,4.93 145.8,2.7 144.21,1.12 95.95,1.12 JP10.30
/IO  (via drill 0.61 pad 1.27)
  Top 0.406: v90.55,55.73 91.5,56.68 v97.22,56.68
  Bottom 0.406: IC16.1 83.88,55.73 v90.55,55.73 | v97.22,56.68 141.67,56.68 148.97,63.98 J1.C11
/LDMEM  (via drill 0.61 pad 1.27)
  Top 0.406: v140.72,10.64 138.49,8.42 v138.49,4.61
  Bottom 0.406: J1.A22 152.78,34.14 152.78,13.82 150.88,11.91 141.99,11.91 v140.72,10.64 | v138.49,4.61 135.95,2.07 109.6,2.07 108.01,3.66 108.01,6.2 109.28,7.47 JP10.15
/MEM2ALUHI
  Bottom 0.406: IC1.2 105.79,80.18 105.79,69.7 94.04,57.95 JP10.27
/MEM2ALULO  (via drill 0.61 pad 1.27)
  Top 0.406: v77.53,88.43 75.95,86.84 IC19.1
  Bottom 0.406: v77.53,88.43 80.39,88.43 81.34,87.48 81.34,86.52 IC19.19 82.93,80.49 96.58,80.49 100.39,76.68 IC1.5 103.89,74.46 103.89,70.97 92.14,59.22 92.14,11.28 JP10.31
/RST  (via drill 0.61 pad 1.27)
  Top 0.406: IC11.2 83.88,10.01 v114.36,10.01
  Bottom 0.406: J1.A20 153.42,42.39 153.42,53.82 152.15,55.09 115.32,55.09 114.36,54.14 IC14.3 114.36,50.33 115.63,49.06 115.63,42.71 120.71,37.63 120.71,9.37 JP10.7 117.54,10.01 v114.36,10.01
ABUS0
  Top 0.406: JP2.1 136.91,37.31 118.81,37.31 IC17.2
  Bottom 0.406: J1.C23 145.8,33.5 144.53,32.23 141.99,32.23 JP2.1
ABUS1
  Top 0.406: J1.A23 153.42,34.77 145.8,34.77 144.53,33.5 JP2.2 138.49,38.26 117.22,38.26 IC17.3
ABUS2
  Top 0.406: JP2.3 138.18,33.5 113.09,33.5 111.82,34.77 IC17.4
  Bottom 0.406: J1.C24 145.8,30.96 144.53,29.69 141.99,29.69 JP2.3
ABUS3
  Top 0.406: J1.A24 153.42,32.23 145.8,32.23 144.53,30.96 JP2.4 141.99,29.69 136.91,29.69 134.05,32.55 112.78,32.55 111.82,33.5 110.55,33.5 109.28,34.77 IC17.5
ABUS4
  Top 0.406: JP2.5 136.59,28.42 133.41,31.6 112.46,31.6 111.51,32.55 110.24,32.55 109.28,33.5 108.01,33.5 106.74,34.77 IC17.6
  Bottom 0.406: J1.C25 145.8,28.42 144.53,27.15 141.99,27.15 JP2.5
ABUS5
  Top 0.406: J1.A25 153.42,29.69 145.8,29.69 144.53,28.42 JP2.6 141.99,27.15 136.27,27.15 132.78,30.64 112.14,30.64 111.19,31.6 109.92,31.6 108.97,32.55 107.7,32.55 106.74,33.5 105.47,33.5 104.2,34.77 IC17.7
ABUS6
  Top 0.406: JP2.7 135.95,25.88 132.14,29.69 111.82,29.69 110.87,30.64 109.6,30.64 108.65,31.6 107.38,31.6 106.43,32.55 105.16,32.55 104.2,33.5 102.93,33.5 101.66,34.77 IC17.8
  Bottom 0.406: J1.C26 145.8,25.88 144.53,24.61 141.99,24.61 JP2.7
ABUS7  (via drill 0.61 pad 1.27)
  Top 0.406: J1.A26 153.42,27.15 145.8,27.15 144.53,25.88 JP2.8 141.99,24.61 v132.14,24.61 | v132.14,40.17 109.28,40.17 106.74,37.63 101.35,37.63 IC17.9
  Bottom 0.406: v132.14,24.61 v132.14,40.17
ABUS8
  Top 0.406: JP2.9 122.94,23.34 122.3,23.98 118.81,23.98 IC18.2
  Bottom 0.406: J1.C27 145.8,23.34 144.53,22.07 141.99,22.07 JP2.9
ABUS9  (via drill 0.61 pad 1.27)
  Top 0.406: J1.A27 153.42,24.61 145.8,24.61 144.53,23.34 JP2.10 141.99,22.07 v124.84,22.07 | v124.84,24.93 117.22,24.93 IC18.3
  Bottom 0.406: v124.84,22.07 v124.84,24.93
ABUS10
  Top 0.406: JP2.11 129.6,20.8 128.97,20.17 113.09,20.17 111.82,21.44 IC18.4
  Bottom 0.406: J1.C28 145.8,20.8 144.53,19.53 141.99,19.53 JP2.11
ABUS11
  Top 0.406: J1.A28 153.42,22.07 145.8,22.07 144.53,20.8 JP2.12 141.99,19.53 129.6,19.53 129.29,19.21 112.78,19.21 111.82,20.17 110.55,20.17 109.28,21.44 IC18.5
ABUS12
  Top 0.406: JP2.13 112.46,18.26 111.51,19.21 110.24,19.21 109.28,20.17 108.01,20.17 106.74,21.44 IC18.6
  Bottom 0.406: J1.C29 145.8,18.26 144.53,16.99 141.99,16.99 JP2.13
ABUS13
  Top 0.406: J1.A29 153.42,19.53 145.8,19.53 144.53,18.26 JP2.14 141.99,16.99 129.6,16.99 129.29,17.31 112.14,17.31 111.19,18.26 109.92,18.26 108.97,19.21 107.7,19.21 106.74,20.17 105.47,20.17 104.2,21.44 IC18.7
ABUS14
  Top 0.406: JP2.15 129.6,15.72 128.97,16.36 111.82,16.36 110.87,17.31 109.6,17.31 108.65,18.26 107.38,18.26 106.43,19.21 105.16,19.21 104.2,20.17 102.93,20.17 101.66,21.44 IC18.8
  Bottom 0.406: J1.C30 145.8,15.72 144.53,14.45 141.99,14.45 JP2.15
ABUS15  (via drill 0.61 pad 1.27)
  Top 0.406: J1.A30 153.42,16.99 145.8,16.99 144.53,15.72 JP2.16 141.67,14.13 v138.18,14.13 | v126.11,26.2 122.62,26.2 122.3,25.88 116.9,25.88 115,23.98 100.71,23.98 99.12,22.39 IC18.9
  Bottom 0.406: v126.11,26.2 v138.18,14.13
ALUBUS0
  Top 0.406: IC4.18 57.21,81.76 55.94,80.49 51.82,80.49 50.55,81.76 R1.2 | IC2.2 26.42,85.89 6.41,85.89 JP3.1
  Bottom 0.406: R1.2 47.05,83.03 31.18,83.03 29.91,84.3 IC2.2
ALUBUS1
  Top 0.406: IC4.17 57.21,79.22 55.94,77.95 51.82,77.95 50.55,79.22 R2.2 47.05,80.49 33.08,80.49 31.81,81.76 IC2.3 25.46,84.3 JP3.2
ALUBUS2
  Top 0.406: IC4.16 57.21,76.68 55.94,75.41 51.82,75.41 50.55,76.68 R3.2 47.05,77.95 33.08,77.95 31.81,79.22 IC2.4 24.19,83.03 6.1,83.03 JP3.3
ALUBUS3
  Top 0.406: IC4.15 57.21,74.14 55.94,72.87 51.82,72.87 50.55,74.14 R4.2 47.05,75.41 33.08,75.41 31.81,76.68 IC2.5 22.92,81.76 JP3.4
ALUBUS4
  Top 0.406: IC4.14 57.21,71.6 55.94,70.33 51.82,70.33 50.55,71.6 R5.2 47.05,72.87 33.08,72.87 31.81,74.14 IC2.6 21.65,80.49 6.1,80.49 JP3.5
ALUBUS5
  Top 0.406: IC4.13 57.21,69.06 55.94,67.79 51.82,67.79 50.55,69.06 R6.2 47.05,70.33 33.08,70.33 31.81,71.6 IC2.7 20.38,79.22 JP3.6
ALUBUS6
  Top 0.406: IC4.12 57.21,66.52 55.94,65.25 51.82,65.25 50.55,66.52 R7.2 47.05,67.79 33.08,67.79 31.81,69.06 IC2.8 19.11,77.95 6.1,77.95 JP3.7
ALUBUS7
  Top 0.406: R8.2 47.05,65.25 33.08,65.25 31.81,66.52 IC2.9 17.84,76.68 JP3.8
  Bottom 0.406: IC4.11 57.21,63.98 55.94,62.71 51.82,62.71 50.55,63.98 R8.2
ALUBUS8
  Top 0.406: IC19.18 81.98,81.76 83.25,80.49 90.55,80.49 91.82,81.76 IC3.18
  Bottom 0.406: IC19.18 76.26,84.62 76.26,89.7 71.5,94.46 27.69,94.46 8.64,75.41 6.1,75.41 JP3.9
ALUBUS9
  Top 0.406: IC19.17 81.98,79.22 83.25,77.95 90.55,77.95 91.82,79.22 IC3.17
  Bottom 0.406: IC19.17 75.31,83.03 75.31,88.11 72.77,90.65 25.78,90.65 9.27,74.14 JP3.10
ALUBUS10
  Top 0.406: IC19.16 81.98,76.68 83.25,75.41 90.55,75.41 91.82,76.68 IC3.16
  Bottom 0.406: IC19.16 74.36,81.44 74.36,87.8 72.45,89.7 26.42,89.7 9.59,72.87 6.1,72.87 JP3.11
ALUBUS11
  Top 0.406: IC19.15 81.98,74.14 83.25,72.87 90.55,72.87 91.82,74.14 IC3.15
  Bottom 0.406: JP3.12 9.91,71.6 27.05,88.75 72.14,88.75 73.41,87.48 73.41,79.86 IC19.15
ALUBUS12
  Top 0.406: IC19.14 81.98,71.6 83.25,70.33 90.55,70.33 91.82,71.6 IC3.14
  Bottom 0.406: IC19.14 74.36,66.84 74.36,62.71 73.09,61.44 22.29,61.44 13.4,70.33 6.1,70.33 JP3.13
ALUBUS13
  Top 0.406: IC19.13 81.98,69.06 83.25,67.79 90.55,67.79 91.82,69.06 IC3.13
  Bottom 0.406: IC19.13 75.63,65.57 75.63,62.71 73.41,60.49 21.34,60.49 12.76,69.06 JP3.14
ALUBUS14
  Top 0.406: IC19.12 81.98,66.52 83.25,65.25 90.55,65.25 91.82,66.52 IC3.12
  Bottom 0.406: IC19.12 76.58,63.98 76.58,62.08 74.04,59.54 20.07,59.54 11.81,67.79 6.1,67.79 JP3.15
ALUBUS15
  Top 0.406: IC19.11 81.98,63.98 83.25,62.71 90.55,62.71 91.82,63.98 IC3.11
  Bottom 0.406: IC19.11 77.85,62.71 77.85,61.44 74.99,58.58 18.8,58.58 10.86,66.52 JP3.16
BUSCLK
  Top 0.406: IC14.11 98.49,48.43 101.66,48.43 | 101.66,48.43 123.89,48.43 128.97,43.35 130.56,43.35 131.51,44.3 131.51,47.15 132.14,47.79 133.73,47.79 135.32,46.2 IC13.3 | IC14.13 101.66,48.43
BUSCLKA
  Bottom 0.406: IC14.9 97.85,51.92 97.85,9.37 JP10.23
BUSCLKB
  Bottom 0.406: IC14.7 100.39,49.38 100.39,6.83 JP10.24
CLK0
  Top 0.406: IC9.12 57.21,49.38 130.24,49.38 | 130.24,49.38 137.86,49.38 | 137.86,49.38 139.13,49.38 140.4,48.11 IC13.5 | IC13.1 130.24,49.38 | IC13.4 137.86,49.38
  Bottom 0.406: IC9.5 53.4,48.11 IC9.12
CLK0A
  Bottom 0.406: IC14.18 114.36,40.17 115.63,38.9 115.63,13.18 111.82,9.37 JP10.13
CLK0B
  Bottom 0.406: IC14.16 108.01,44.3 108.01,7.47 106.74,6.2 JP10.18
CLK0C
  Bottom 0.406: IC14.14 102.93,44.3 102.93,9.37 JP10.19
CLK0D  (via drill 0.61 pad 1.27)
  Top 0.406: v105.47,42.39 102.3,42.39 IC14.12
  Bottom 0.406: v105.47,42.39 105.47,9.37 JP10.17
CLK1
  Bottom 0.406: IC14.5 110.55,51.92 110.55,4.29 110.87,3.98 115.32,3.98 JP10.10
DBUS0
  Top 0.406: J1.C3 149.29,83.99 145.48,83.99 144.53,83.03 141.99,83.03 JP1.1 R9.2 135.32,85.57 118.49,85.57 IC6.2 115.95,85.57 91.82,85.57 90.55,84.3 IC3.2 85.15,85.57 54.99,85.57 IC4.2
DBUS1
  Top 0.406: J1.C4 149.29,81.44 145.48,81.44 144.53,80.49 141.99,80.49 JP1.3 R10.2 135.32,83.03 118.49,83.03 IC6.3 115.95,83.03 91.82,83.03 90.55,81.76 IC3.3 83.25,81.76 81.98,83.03 57.21,83.03 55.94,81.76 IC4.3
DBUS2
  Top 0.406: J1.C5 149.29,78.91 145.48,78.91 144.53,77.95 141.99,77.95 JP1.5 R11.2 135.32,80.49 118.49,80.49 IC6.4 115.95,80.49 91.82,80.49 90.55,79.22 IC3.4 83.25,79.22 81.98,80.49 57.21,80.49 55.94,79.22 IC4.4
DBUS3
  Top 0.406: J1.C6 149.29,76.36 145.48,76.36 144.53,75.41 141.99,75.41 JP1.7 R12.2 135.32,77.95 118.49,77.95 IC6.5 115.95,77.95 91.82,77.95 90.55,76.68 IC3.5 83.25,76.68 81.98,77.95 57.21,77.95 55.94,76.68 IC4.5
DBUS4
  Top 0.406: J1.C7 149.29,73.83 145.48,73.83 144.53,72.87 141.99,72.87 JP1.9 R13.2 135.32,75.41 118.49,75.41 IC6.6 115.95,75.41 91.82,75.41 90.55,74.14 IC3.6 83.25,74.14 81.98,75.41 57.21,75.41 55.94,74.14 IC4.6
DBUS5
  Top 0.406: J1.C8 149.29,71.29 145.48,71.29 144.53,70.33 141.99,70.33 JP1.11 R14.2 135.32,72.87 118.49,72.87 IC6.7 115.63,70.02 99.76,70.02 96.9,72.87 91.82,72.87 90.55,71.6 IC3.7 83.25,71.6 81.98,72.87 57.21,72.87 55.94,71.6 IC4.7
DBUS6
  Top 0.406: J1.C9 149.29,68.74 145.48,68.74 144.53,67.79 141.99,67.79 JP1.13 R15.2 135.32,70.33 118.49,70.33 IC6.8 97.54,69.06 96.27,70.33 91.82,70.33 90.55,69.06 IC3.8 83.25,69.06 81.98,70.33 57.21,70.33 55.94,69.06 IC4.8
DBUS7
  Top 0.406: J1.C10 149.29,66.21 145.48,66.21 144.53,65.25 141.99,65.25 JP1.15 R16.2 135.32,67.79 118.49,67.79 IC6.9 115.95,67.79 91.82,67.79 90.55,66.52 IC3.9 83.25,66.52 81.98,67.79 71.5,67.79 | 71.5,67.79 57.21,67.79 55.94,66.52 IC4.9 | IC19.8 71.5,67.79
  Bottom 0.406: IC19.2 IC19.3 IC19.4 IC19.5 IC19.6 IC19.7 IC19.8 IC19.9
GND  (via drill 0.61 pad 1.27)
  Bottom 0.406: LED1.K 8.95,46.56 S1.4
  other vias: 96.27,39.85 90.55,22.71
  pour Top (isolate 0.61): 0.06,99.86 160.08,99.86 160.08,-0.15 0.06,-0.15
  pour Bottom (isolate 0.61): 0.06,99.86 160.08,99.86 160.08,-0.15 0.06,-0.15
IRQ0
  Top 0.406: J1.A3 153.42,85.57 148.65,85.57 148.34,85.25 145.48,85.25 144.53,84.3 JP1.2
IRQ1
  Top 0.406: J1.A4 153.42,83.03 148.65,83.03 148.34,82.72 145.48,82.72 144.53,81.76 JP1.4
IRQ2
  Top 0.406: J1.A5 153.42,80.49 148.65,80.49 148.34,80.18 145.48,80.18 144.53,79.22 JP1.6
IRQ3
  Top 0.406: J1.A6 153.42,77.95 148.65,77.95 148.34,77.63 145.48,77.63 144.53,76.68 JP1.8
IRQ4
  Top 0.406: J1.A7 153.42,75.41 148.65,75.41 148.34,75.1 145.48,75.1 144.53,74.14 JP1.10
IRQ5
  Top 0.406: J1.A8 153.42,72.87 148.65,72.87 148.34,72.55 145.48,72.55 144.53,71.6 JP1.12
IRQ6
  Top 0.406: J1.A9 153.42,70.33 148.65,70.33 148.34,70.02 145.48,70.02 144.53,69.06 JP1.14
IRQ7
  Top 0.406: J1.A10 153.42,67.79 148.65,67.79 148.34,67.47 145.48,67.47 144.53,66.52 JP1.16
MEMSEG
  Bottom 0.406: J1.A21 151.83,35.72 151.83,15.72 150.56,14.45 146.11,14.45 145.16,13.5 141.03,13.5 134.37,6.83 113.09,6.83 JP10.14
N$1
  Bottom 0.406: IC1.3 99.12,84.3 IC3.19
N$2
  Bottom 0.406: IC1.6 100.39,72.87 76.9,72.87 73.41,69.38 73.41,63.03 72.77,62.39 69.28,62.39 66.74,64.94 66.74,81.76 64.2,84.3 IC4.19
N$3
  Top 0.406: R1.1 IC2.18
N$4
  Top 0.406: R2.1 IC2.17
N$5
  Top 0.406: IC2.16 R3.1
N$6
  Top 0.406: IC2.15 R4.1
N$7
  Top 0.406: IC2.14 R5.1
N$8
  Top 0.406: IC2.13 R6.1
N$9
  Top 0.406: IC2.12 R7.1
N$10
  Top 0.406: IC2.11 R8.1
N$11
  Bottom 0.406: R9.1 126.43,81.76 IC6.18
N$12
  Bottom 0.406: R10.1 126.43,79.22 IC6.17
N$13
  Bottom 0.406: R11.1 126.43,76.68 IC6.16
N$14
  Bottom 0.406: R12.1 126.43,74.14 IC6.15
N$15
  Bottom 0.406: R13.1 126.43,71.6 IC6.14
N$16
  Bottom 0.406: R15.1 126.43,66.52 IC6.12
N$17
  Bottom 0.406: R16.1 126.43,63.98 IC6.11
N$18
  Bottom 0.406: R14.1 126.43,69.06 IC6.13
N$19
  Top 0.406: S1.1 S1.2
  Bottom 0.406: S1.1 21.65,22.28 21.65,5.88 22.61,4.93 IC12.1
N$20
  Top 0.406: IC10.11 69.91,48.11 IC10.3 58.48,48.11 IC9.11 53.4,48.11 IC9.3
  Bottom 0.406: IC9.3 40.7,55.73 OSC1.8
N$21
  Top 0.406: R18.1 LED1.A
N$22
  Top 0.406: IC9.8 52.13,41.76 47.05,41.76 46.1,42.71 46.1,49.69 47.05,50.65 IC9.2
N$23  (via drill 0.61 pad 1.27)
  Top 0.406: IC14.17 104.84,38.58 94.68,38.58 91.5,35.41 v64.52,35.41
  Bottom 0.406: v64.52,35.41 55.94,26.84 55.94,6.2 IC15.5
N$24
  Bottom 0.406: IC12.6 30.54,14.45 32.45,14.45 R19.1 37.53,14.45 41.02,14.45 43.24,12.23 43.24,8.74 IC15.2
N$25  (via drill 0.61 pad 1.27)
  Top 0.406: IC10.8 69.91,40.49 v67.37,40.49
  Bottom 0.406: v67.37,40.49 66.1,41.76 63.56,41.76 62.93,42.39 62.93,48.74 IC10.2
N$26
  Top 0.406: IC14.8 104.2,50.65 106.74,50.65 | 106.74,50.65 111.82,50.65 | 111.82,50.65 116.9,50.65 | 116.9,50.65 121.03,50.65 122.62,52.24 124.84,52.24 126.43,50.65 143.26,50.65 145.48,52.87 IC13.8 | IC14.6 106.74,50.65 | IC14.2 116.9,50.65 | IC14.4 111.82,50.65
N$27
  Bottom 0.406: IC11.13 81.34,5.24 85.79,9.69 85.79,48.74 82.61,51.92 69.91,51.92 67.37,54.46 61.34,54.46 58.8,51.92 50.86,51.92 49.59,53.19 IC9.1
N$28
  Top 0.406: C1.+ R17.1
  Bottom 0.406: R17.1 26.73,39.22 67.69,39.22 70.23,41.76 74.36,41.76 80.71,48.11 IC16.3
N$29
  Top 0.406: IC13.10 IC13.9 142.94,53.82 144.84,55.73 146.11,55.73 147.7,54.14 147.7,50.33 IC13.6
N$30  (via drill 0.61 pad 1.27)
  Top 0.406: IC12.7 29.59,9.05 45.78,9.05 49.59,5.24 IC15.3 | v58.48,36.04 58.48,37.95 IC9.9 57.21,41.76 74.68,41.76 79.76,46.84 91.19,46.84 96.9,41.12 106.11,41.12 106.74,41.76 IC14.15 108.65,47.47 123.57,47.47 128.65,42.39 130.87,42.39 132.78,44.3 IC13.2
  Bottom 0.406: v58.48,36.04 48.32,25.88 35.62,25.88 26.1,16.36 IC12.7
N$31
  Bottom 0.406: IC10.5 69.91,48.11 IC10.12
N$32
  Bottom 0.406: IC11.1 81.34,10.01 78.49,10.01 77.53,10.96 77.53,36.04 73.09,40.49 IC10.9
N$33
  Top 0.406: IC11.14 78.8,10.01 IC11.3
  Bottom 0.406: IC11.3 84.52,18.26 84.52,48.74 82.61,50.65 IC16.2
N$34
  Bottom 0.406: IC16.4 IC16.5
N$35
  Top 0.406: IC9.13 57.21,51.92 71.18,51.92 IC10.13
  Bottom 0.406: IC16.6 83.57,42.71 83.57,48.43 82.61,49.38 76.26,49.38 74.99,50.65 IC10.13
RBUS0  (via drill 0.61 pad 1.27)
  Top 0.406: IC17.18 111.51,24.93 32.13,24.93 31.5,24.3 v28.64,24.3 | v28.64,35.09 6.41,35.09 JP4.1
  Bottom 0.406: v28.64,24.3 v28.64,35.09
RBUS1
  Top 0.406: IC17.17 109.92,29.69 109.28,29.69 108.33,30.64 107.06,30.64 106.11,31.6 104.84,31.6 103.89,32.55 102.62,32.55 101.66,33.5 JP4.2
RBUS2
  Top 0.406: IC17.16 107.38,29.69 106.74,29.69 105.79,30.64 104.52,30.64 103.57,31.6 102.3,31.6 101.35,32.55 13.4,32.55 13.08,32.23 6.1,32.23 JP4.3
RBUS3
  Top 0.406: IC17.15 104.84,29.69 104.2,29.69 103.25,30.64 101.98,30.64 101.03,31.6 13.72,31.6 13.08,30.96 JP4.4
RBUS4
  Top 0.406: IC17.14 102.3,29.69 101.66,29.69 100.71,30.64 14.03,30.64 13.08,29.69 6.1,29.69 JP4.5
RBUS5
  Top 0.406: IC17.13 99.76,29.69 14.35,29.69 13.08,28.42 JP4.6
RBUS6  (via drill 0.61 pad 1.27)
  Top 0.406: IC17.12 97.22,25.88 v15.3,25.88
  Bottom 0.406: v15.3,25.88 14.03,27.15 6.1,27.15 JP4.7
RBUS7
  Top 0.406: IC17.11 14.67,27.79 12.76,25.88 JP4.8
RBUS8  (via drill 0.61 pad 1.27)
  Top 0.406: IC18.18 111.19,11.28 v88.33,11.28 | JP4.9 6.1,24.61 11.81,24.61 13.72,22.71 v88.33,22.71
  Bottom 0.406: v88.33,11.28 v88.33,22.71
RBUS9
  Top 0.406: IC18.17 111.82,15.09 110.55,16.36 109.28,16.36 108.33,17.31 107.06,17.31 106.11,18.26 104.84,18.26 103.89,19.21 102.62,19.21 101.66,20.17 13.4,20.17 10.22,23.34 JP4.10
RBUS10
  Top 0.406: IC18.16 109.28,15.09 108.01,16.36 106.74,16.36 105.79,17.31 104.52,17.31 103.57,18.26 102.3,18.26 101.35,19.21 13.08,19.21 10.22,22.07 6.1,22.07 JP4.11
RBUS11
  Top 0.406: IC18.15 106.74,14.77 105.16,16.36 104.2,16.36 103.25,17.31 101.98,17.31 101.03,18.26 12.76,18.26 10.22,20.8 JP4.12
RBUS12
  Top 0.406: IC18.14 104.2,15.09 102.93,16.36 101.66,16.36 100.71,17.31 12.45,17.31 10.22,19.53 6.1,19.53 JP4.13
RBUS13
  Top 0.406: IC18.13 101.66,15.09 100.39,16.36 12.13,16.36 10.22,18.26 JP4.14
RBUS14
  Top 0.406: IC18.12 97.22,12.55 92.46,12.55 90.55,14.45 12.13,14.45 11.49,13.82 6.73,13.82 JP4.15
RBUS15
  Top 0.406: IC18.11 95.63,15.4 7.68,15.4 JP4.16
RST  (via drill 0.61 pad 1.27)
  Top 0.406: v66.42,3.66 67.37,2.7 116.59,2.7 118.17,4.29 118.17,6.83 JP10.9 | v62.93,3.66 61.66,3.66 61.02,3.02 58.48,3.02 57.21,4.29 IC15.6
  Bottom 0.406: v66.42,3.66 v62.93,3.66

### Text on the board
Top: #0
_tsilk: VCC2 | GND1 | IC2 | IC4 | IC19 | IC3 | IC1 | IC6 | JP3 | 74LS08N | JP1 | 74LS541N | 74LS245N | 74LS541N | 74LS245N | 74LS541N | 10k | 10k | OSC1 | LED1 | IC9 | IC10 | IC16 | IC14 | 74LS74N | 74LS74N | 74LS14N | 16.000MHz | 400 | 74LS244N | 74LS32N | R18 | IC13 | 10u | R17 | S1 | 10k | C1 | JP4 | IC17 | JP2 | 74LS541N | IC18 | 74LS541N | IC11 | R19 | GND2 | 4k | 74LS73N | VCC1 | 10u | MAX1232 | 74LS74N | IC12 | IC15 | JP10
